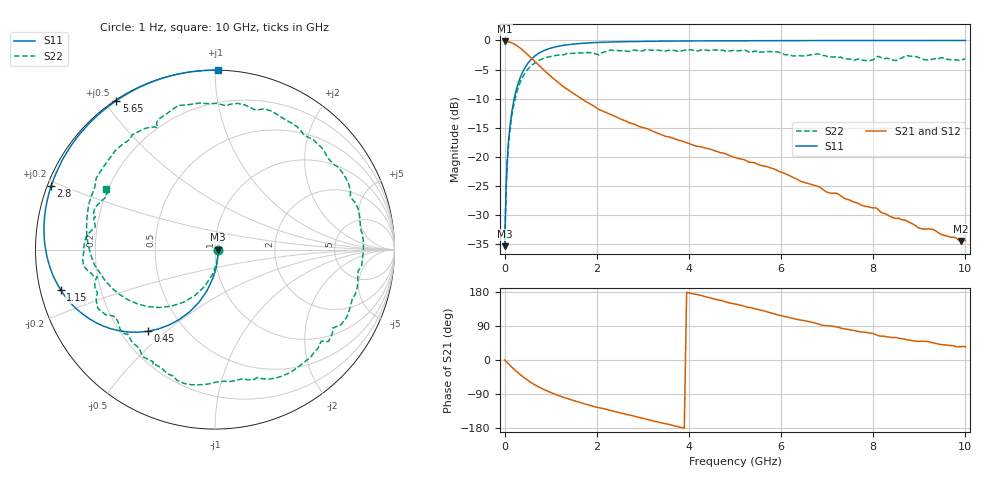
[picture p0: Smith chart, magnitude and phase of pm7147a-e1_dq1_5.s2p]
# GHz S DB R 50
! S-Parameters data
! Freq  dbS11  angS11  dbS21  angS21  dbS12  angS12  dbS22  angS22
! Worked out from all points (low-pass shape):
!   279 points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, 1 Hz to 10 GHz, reference 50 ohm
!   highest |S21| = -0.15 dB at 199.5 Hz (marker M1); lowest = -34.5 dB at 9.9 GHz (marker M2)
!   |S21| within 3 dB of the highest: start of sweep to 593 MHz
!   lowest |S11| = -35.4 dB at 39.8 Hz (marker M3), VSWR 1.03, Z = 51.7 - j6.4e-06 ohm
!   |S11| at or under -10 dB: start of sweep to 208.5 MHz
!   |S22| runs from -35.4 to -1.6 dB; largest |S21 - S12| = 0
!   S11 on the Smith chart (normalised r, x): 1 Hz: 1.03, -0.00; 450 MHz: 0.31, -0.43; 1.15 GHz: 0.06, -0.13; 2.8 GHz: 0.01, +0.19; 5.65 GHz: 0.00, +0.54; 10 GHz: 0.00, +1.02
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1e-09  -35.39 -0.0  -0.15 -0.0  -0.15 -0.0  -35.39 -0.0
3.98e-08  -35.39 -0.0  -0.15 -0.0  -0.15 -0.0  -35.39 -0.0
1.995e-07  -35.39 -0.0  -0.15 -0.0  -0.15 -0.0  -35.39 -0.0
0.03981072  -23.64 -78.8  -0.17 -4.8  -0.17 -4.8  -24.28 -79.2
0.1  -15.98 -94.1  -0.26 -12.0  -0.26 -12.0  -16.65 -97.3
0.25  -8.57 -112.0  -0.82 -29.2  -0.82 -29.2  -9.31 -120.9
0.45  -4.57 -129.5  -2.07 -49.1  -2.07 -49.1  -5.52 -145.3
0.8  -1.94 -151.2  -4.71 -74.8  -4.71 -74.8  -3.22 -176.7
1.15  -1.02 -165.4  -7.13 -92.9  -7.13 -92.9  -2.53 159.9
1.7  -0.49 179.3  -10.17 -114.5  -10.17 -114.5  -2.17 130.1
2.3  -0.27 167.2  -12.72 -133.0  -12.72 -133.0  -1.63 104.2
2.8  -0.18 158.8  -14.38 -148.0  -14.38 -148.0  -1.68 81.3
3.35  -0.13 150.7  -16.04 -164.4  -16.04 -164.4  -1.69 56.3
4.3  -0.08 138.3  -18.38 169.1  -18.38 169.1  -1.62 15.3
5.05  -0.05 129.8  -20.27 146.5  -20.27 146.5  -1.80 -19.7
5.65  -0.04 123.5  -21.61 128.8  -21.61 128.8  -1.93 -48.0
6.7  -0.02 113.5  -24.89 98.6  -24.89 98.6  -2.40 -96.9
7.3  -0.01 108.3  -26.74 83.8  -26.74 83.8  -2.85 -124.1
8.35  -0.01 100.1  -30.20 60.2  -30.20 60.2  -3.14 -164.1
8.75  -0.01 97.2  -31.13 52.8  -31.13 52.8  -2.63 -176.3
9.9  -0.00 89.7  -34.48 35.3  -34.48 35.3  -3.39 152.4
10  -0.00 89.1  -34.41 34.9  -34.41 34.9  -3.14 151.1
